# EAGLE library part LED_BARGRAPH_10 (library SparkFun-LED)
10-Segment LED Bar Graph SFE part numbers: COM-09935 (red, Vf = 2.1V, Ifmax = 20mA) COM-09936 (yellow, Vf = 2.1V, Ifmax = 20mA) COM-09937 (blue, Vf = 3.4V, Ifmax = 20mA) COM-09938 (green, Vf = 3.4V, Ifmax = 20mA)
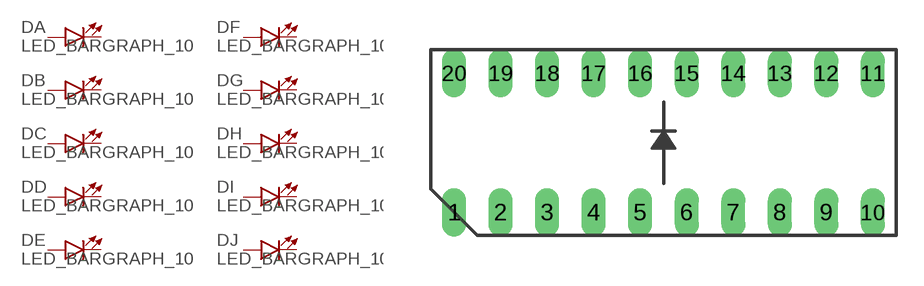
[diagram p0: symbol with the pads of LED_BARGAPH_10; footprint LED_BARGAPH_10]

Designator prefix D; gates A=LED_BARGRAPH_10 B=LED_BARGRAPH_10 C=LED_BARGRAPH_10 D=LED_BARGRAPH_10 E=LED_BARGRAPH_10 F=LED_BARGRAPH_10 G=LED_BARGRAPH_10 H=LED_BARGRAPH_10 I=LED_BARGRAPH_10 J=LED_BARGRAPH_10

## LED_BARGRAPH_10  [LED_BARGAPH_10]
1  A:A  pas
2  B:A  pas
3  C:A  pas
4  D:A  pas
5  E:A  pas
6  F:A  pas
7  G:A  pas
8  H:A  pas
9  I:A  pas
10  J:A  pas
11  J:C  pas
12  I:C  pas
13  H:C  pas
14  G:C  pas
15  F:C  pas
16  E:C  pas
17  D:C  pas
18  C:C  pas
19  B:C  pas
20  A:C  pas

## Footprint LED_BARGAPH_10 (pad centres in mm)
Dual In Line Package
drill 0.813 long: 1 -11.43,-3.81; 2 -8.89,-3.81; 3 -6.35,-3.81; 4 -3.81,-3.81; 5 -1.27,-3.81; 6 1.27,-3.81; 7 3.81,-3.81; 8 6.35,-3.81; 9 8.89,-3.81; 10 11.43,-3.81; 11 11.43,3.81; 12 8.89,3.81; 13 6.35,3.81; 14 3.81,3.81; 15 1.27,3.81; 16 -1.27,3.81; 17 -3.81,3.81; 18 -6.35,3.81; 19 -8.89,3.81; 20 -11.43,3.81

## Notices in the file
Licensing: CC v3.0 Share-Alike You are welcome to use this library for commercial purposes.
